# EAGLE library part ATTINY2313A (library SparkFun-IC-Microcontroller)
ATTINY2313A 2kB 20MHz I2C/SPI/UART Datasheet SparkFun Products SparkFun Wake on Shake (SEN-11447)
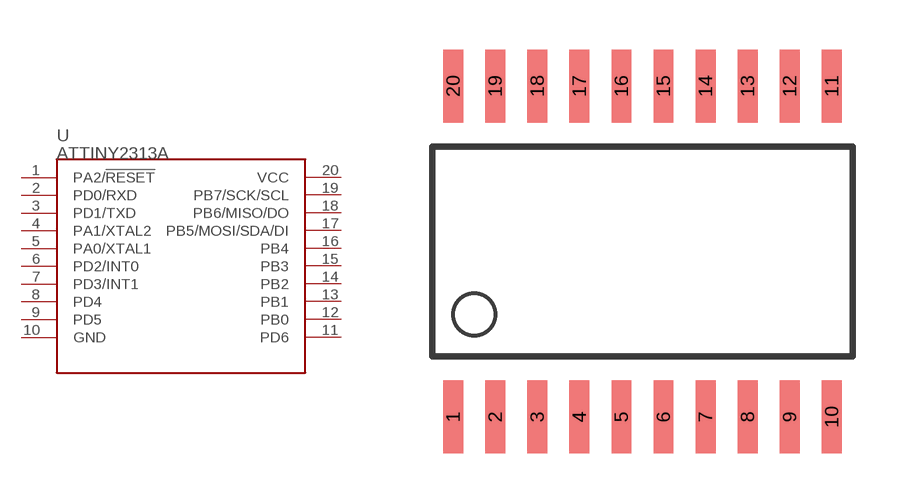
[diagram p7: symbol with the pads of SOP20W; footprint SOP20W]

Designator prefix U

## ATTINY2313A (PROD_ID: IC-11305; VALUE: ATTINY2313A)  [SOP20W]
1  PA2/!RESET
2  PD0/RXD
3  PD1/TXD
4  PA1/XTAL2
5  PA0/XTAL1
6  PD2/INT0
7  PD3/INT1
8  PD4
9  PD5
10  GND
11  PD6
12  PB0
13  PB1
14  PB2
15  PB3
16  PB4
17  PB5/MOSI/SDA/DI
18  PB6/MISO/DO
19  PB7/SCK/SCL
20  VCC

## Footprint SOP20W (pad centres in mm)
SMALL OUTLINE PACKAGE
smd 0.6 x 2.2: 1 -5.715,-5; 2 -4.445,-5; 3 -3.175,-5; 4 -1.905,-5; 5 -0.635,-5; 6 0.635,-5; 7 1.905,-5; 8 3.175,-5; 9 4.445,-5; 10 5.715,-5; 11 5.715,5; 12 4.445,5; 13 3.175,5; 14 1.905,5; 15 0.635,5; 16 -0.635,5; 17 -1.905,5; 18 -3.175,5; 19 -4.445,5; 20 -5.715,5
